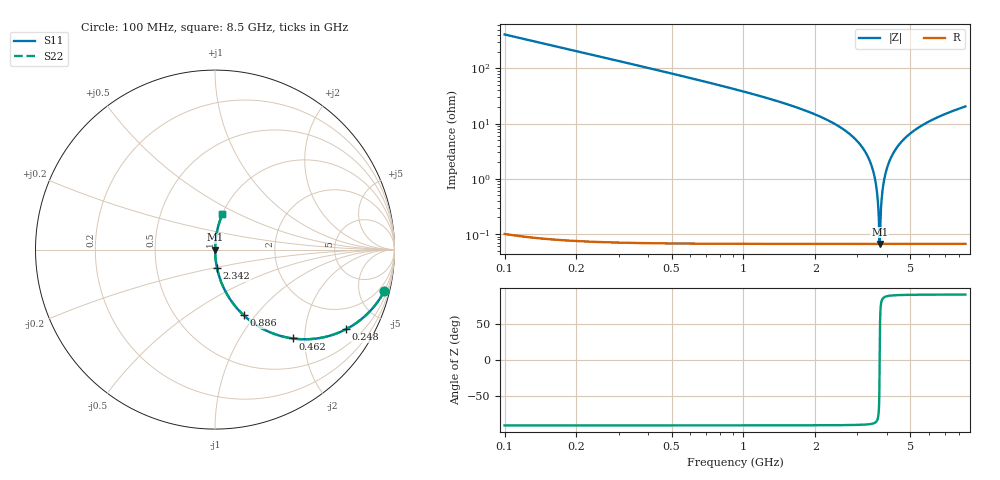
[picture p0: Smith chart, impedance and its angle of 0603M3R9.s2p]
! Created Wed Apr 18 15:37:32 2012
# hz S ma R 50
! 2 Port Network Data from SP1.SP block
! freq  magS11  angS11  magS21  angS21  magS12  angS12  magS22  angS22
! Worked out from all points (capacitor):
!   8401 points, 100 MHz to 8.5 GHz, reference 50 ohm
!   read as one part in series: C = 3.88 pF near 142 MHz
!   lowest |Z| = 66.2 mohm at 3.719 GHz (marker M1)
!   series resonance near 3.719 GHz, so ESL is about 470 pH
!   S11 on the Smith chart (normalised r, x): 100 MHz: 1.00, -8.20; 248 MHz: 1.00, -3.29; 462 MHz: 1.00, -1.75; 886 MHz: 1.00, -0.87; 2.342 GHz: 1.00, -0.21; 8.5 GHz: 1.00, +0.41
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1e8  0.9715 -13.7  0.237 76.3  0.237 76.3  0.9715 -13.7
2.48e8  0.8546 -31.3  0.519 58.7  0.519 58.7  0.8546 -31.3
4.62e8  0.6579 -48.8  0.7526 41.1  0.7526 41.1  0.6579 -48.8
8.86e8  0.4 -66.3  0.9159 23.6  0.9159 23.6  0.4 -66.3
1.5e9  0.2231 -76.9  0.9742 12.9  0.9742 12.9  0.2231 -76.9
2.342e9  0.105 -83.6  0.9938 6.0  0.9938 6.0  0.105 -83.6
2.9e9  0.05533 -86.1  0.9978 3.2  0.9978 3.2  0.05533 -86.1
3.257e9  0.02932 -87.0  0.9989 1.7  0.9989 1.7  0.02932 -87.0
3.489e9  0.01409 -86.5  0.9992 0.8  0.9992 0.8  0.01409 -86.5
3.615e9  0.006284 -83.6  0.9993 0.4  0.9993 0.4  0.006284 -83.6
3.653e9  0.003998 -80.3  0.9993 0.2  0.9993 0.2  0.003998 -80.3
3.693e9  0.001677 -66.7  0.9993 0.1  0.9993 0.1  0.001677 -66.7
3.719e9  0.0006613 0.5  0.9993 -0.0  0.9993 -0.0  0.0006613 0.5
3.745e9  0.001678 66.7  0.9993 -0.1  0.9993 -0.1  0.001678 66.7
3.812e9  0.005493 82.8  0.9993 -0.3  0.9993 -0.3  0.005493 82.8
3.901e9  0.01057 85.8  0.9993 -0.6  0.9993 -0.6  0.01057 85.8
4.062e9  0.01949 86.9  0.9991 -1.1  0.9991 -1.1  0.01949 86.9
4.3e9  0.03212 87.0  0.9988 -1.8  0.9988 -1.8  0.03212 87.0
4.857e9  0.05949 86.0  0.9976 -3.4  0.9976 -3.4  0.05949 86.0
5.7e9  0.09664 84.1  0.9947 -5.5  0.9947 -5.5  0.09664 84.1
7.1e9  0.1511 81.1  0.9879 -8.7  0.9879 -8.7  0.1511 81.1
8.5e9  0.1999 78.3  0.9792 -11.5  0.9792 -11.5  0.1999 78.3
